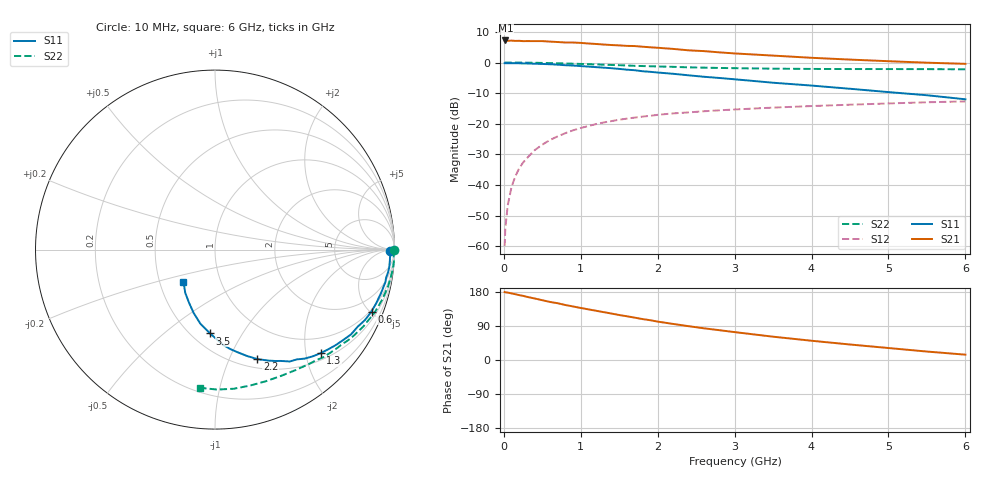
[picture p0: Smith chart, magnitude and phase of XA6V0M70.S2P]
! SIEMENS Discrete & RF Semiconductors
! BFY180
! Si NPN RF Bipolar Junction Transistor in MICRO-X
! VCE = 6 V  IC = 0.7 mA
! Common Emitter S-Parameters:  May  1997
# GHz  S  MA  R  50
!  f  S11  S21  S12  S22
! GHz  MAG  ANG  MAG  ANG  MAG  ANG  MAG  ANG
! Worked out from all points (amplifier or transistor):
!   36 points, 10 MHz to 6 GHz, reference 50 ohm
!   highest |S21| = 7.2 dB at 20 MHz (marker M1)
!   |S21| within 3 dB of that: start of sweep to 2.304 GHz
!   unconditionally stable (mu >= 1): 5.137 GHz to end of sweep
!   at 250 MHz: K = 0.06, MSG = 19.8 dB, |S12| = -32.7 dB
!   at 1.4 GHz: K = 0.42, MSG = 12.4 dB, |S12| = -19.1 dB
!   at 6 GHz: K = 1.03, MAG = 5.1 dB, |S12| = -12.7 dB
!   S11 on the Smith chart (normalised r, x): 10 MHz: 80, -17; 600 MHz: 0.89, -5.09; 1.3 GHz: 0.64, -2.30; 2.2 GHz: 0.60, -1.28; 3.5 GHz: 0.61, -0.73; 6 GHz: 0.66, -0.25
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0.01  0.9763 -0.3  2.273 179.4  0.001 87.4  0.9993 -0.2
0.02  0.9748 -0.7  2.294 178.7  0.002 103.4  0.9999 -0.5
0.05  0.9761 -1.6  2.261 177.9  0.0046 90.3  0.9979 -1.2
0.1  0.9763 -3.7  2.281 175.7  0.0093 84.8  0.996 -2.4
0.15  0.9759 -5.7  2.255 173.6  0.0139 87.1  0.9991 -3.6
0.2  0.9731 -7.3  2.262 171.2  0.0187 84.6  0.9978 -4.8
0.4  0.9569 -14.4  2.239 162.4  0.0369 79.8  0.9908 -9.5
0.5  0.9474 -18.1  2.239 157.8  0.0456 76.6  0.9855 -12.0
0.6  0.9378 -21.6  2.197 153.2  0.0543 74.0  0.9789 -14.2
0.9  0.8932 -31.9  2.124 141.3  0.0781 66.0  0.9575 -21.0
1.1  0.8579 -38.3  2.047 133.6  0.0918 61.2  0.9391 -25.1
1.3  0.8243 -44.4  1.967 126.2  0.1051 56.8  0.9214 -29.2
1.7  0.7493 -56.3  1.859 111.8  0.126 49.1  0.8832 -36.5
2  0.6869 -64.2  1.742 101.3  0.1398 44.2  0.8629 -41.6
2.2  0.6546 -68.8  1.67 95.2  0.1476 41.0  0.8507 -44.8
2.6  0.5855 -77.6  1.537 83.7  0.1599 35.8  0.8253 -50.5
2.8  0.5596 -81.4  1.467 78.7  0.1657 33.5  0.8155 -53.3
3.5  0.4678 -93.4  1.298 61.5  0.1835 26.2  0.7941 -62.4
4  0.4205 -101.2  1.195 50.8  0.1945 21.5  0.7862 -68.9
4.5  0.3728 -108.6  1.117 40.9  0.2047 17.3  0.7824 -75.5
5.5  0.2921 -124.6  0.994 22.3  0.2242 8.7  0.7799 -89.2
6  0.2509 -134.4  0.952 14.1  0.2318 4.4  0.7744 -96.1
